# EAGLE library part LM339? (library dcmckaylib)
Quad Comparator. Same as LM239/2901.
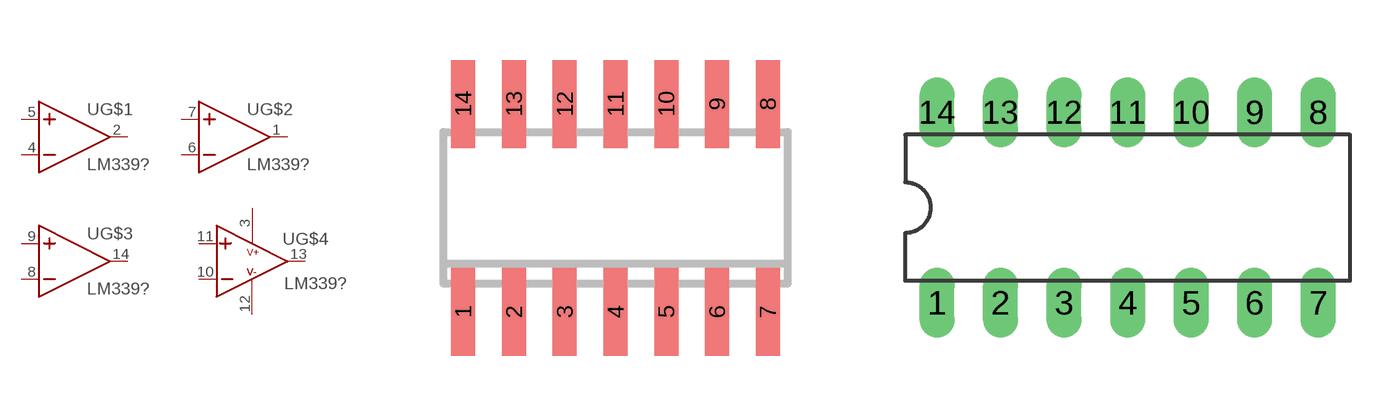
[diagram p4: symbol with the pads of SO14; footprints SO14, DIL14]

Designator prefix U; gates G$1=OPAMP G$2=OPAMP G$3=OPAMP G$4=OPAMP2

## LM339D  [SO14]
1  G$2:OUT  out
2  G$1:OUT  out
3  G$4:V+  pwr
4  G$1:IN-  in
5  G$1:IN+  in
6  G$2:IN-  in
7  G$2:IN+  in
8  G$3:IN-  in
9  G$3:IN+  in
10  G$4:IN-  in
11  G$4:IN+  in
12  G$4:V-  pwr
13  G$4:OUT  out
14  G$3:OUT  out

## LM339N  [DIL14]
Pads as for SO14

## Footprint SO14 (pad centres in mm)
Small Outline Package 14
smd 0.6 x 2.2: 1 -3.81,-2.6; 2 -2.54,-2.6; 3 -1.27,-2.6; 4 0,-2.6; 5 1.27,-2.6; 6 2.54,-2.6; 7 3.81,-2.6; 8 3.81,2.6; 9 2.54,2.6; 10 1.27,2.6; 11 0,2.6; 12 -1.27,2.6; 13 -2.54,2.6; 14 -3.81,2.6

## Footprint DIL14 (pad centres in mm)
Dual In Line Package
drill 0.889 long: 1 -7.62,-3.81; 2 -5.08,-3.81; 3 -2.54,-3.81; 4 0,-3.81; 5 2.54,-3.81; 6 5.08,-3.81; 7 7.62,-3.81; 8 7.62,3.81; 9 5.08,3.81; 10 2.54,3.81; 11 0,3.81; 12 -2.54,3.81; 13 -5.08,3.81; 14 -7.62,3.81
